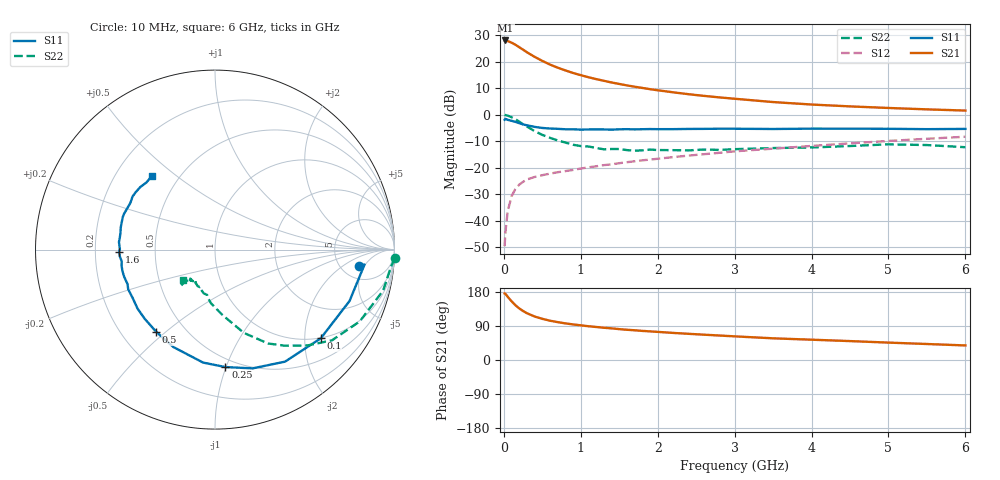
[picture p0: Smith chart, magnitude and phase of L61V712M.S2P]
!  INFINEON TECHNOLOGIES Small Signal Semiconductors
! BFR380L3 , Si-NPN RF-Transistor in TSLP-3-1
!  Vce=1.75 V,  Ic=12.5 mA
! Common Emitter S-Parameters:  07. March 2005
#  GHz  S  MA  R  50
! f  S11  S21  S12  S22
! GHz  Mag  Ang  Mag  Ang  Mag  Ang  Mag  Ang
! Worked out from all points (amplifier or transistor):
!   36 points, 10 MHz to 6 GHz, reference 50 ohm
!   highest |S21| = 28.1 dB at 20 MHz (marker M1)
!   |S21| within 3 dB of that: start of sweep to 224.2 MHz
!   unconditionally stable (mu >= 1): 2.034 GHz to 4.841 GHz
!   at 250 MHz: K = 0.29, MSG = 24.9 dB, |S12| = -25.3 dB
!   at 1.4 GHz: K = 0.91, MSG = 15.5 dB, |S12| = -18.7 dB
!   at 6 GHz: K = 0.97, MSG = 4.9 dB, |S12| = -8.3 dB
!   S11 on the Smith chart (normalised r, x): 10 MHz: 7.23, -3.80; 100 MHz: 0.99, -2.39; 250 MHz: 0.43, -1.00; 500 MHz: 0.35, -0.47; 1.6 GHz: 0.30, -0.01; 6 GHz: 0.36, +0.41
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0.01  0.805 -6.6  25.27 175.6  0.0033 84.4  1.002 -2.8
0.02  0.8373 -5.7  25.29 174.9  0.0059 91.9  0.9845 -5.7
0.05  0.8024 -20.9  24.63 166.9  0.015 81.4  0.9642 -13.7
0.1  0.7691 -40.0  23 155.1  0.0288 70.4  0.9002 -26.4
0.15  0.7361 -58.0  21.05 144.6  0.0397 63.4  0.8248 -37.8
0.2  0.6942 -72.4  18.87 136.1  0.0479 59.1  0.7424 -46.0
0.25  0.6571 -84.9  16.94 129.3  0.0542 54.0  0.6608 -54.1
0.3  0.633 -96.0  15.13 123.5  0.06 51.5  0.6011 -60.5
0.4  0.5903 -113.1  12.41 114.7  0.0668 48.7  0.491 -70.9
0.5  0.5632 -125.5  10.4 108.7  0.0723 47.5  0.4171 -77.2
0.6  0.5496 -135.4  8.864 103.7  0.0773 47.1  0.3667 -83.5
0.7  0.5424 -142.7  7.751 100.0  0.0822 48.0  0.3273 -89.1
0.9  0.5318 -155.4  6.144 93.9  0.0909 49.5  0.2713 -98.4
1.1  0.5279 -163.0  5.11 89.1  0.1018 51.5  0.2515 -104.6
1.4  0.5236 -172.7  4.07 83.5  0.1158 54.1  0.2257 -112.1
1.6  0.5345 -178.6  3.585 79.8  0.127 55.0  0.215 -119.9
2.2  0.535 169.9  2.656 71.5  0.1586 57.9  0.2146 -124.8
2.8  0.5449 160.4  2.129 64.6  0.1911 59.7  0.2171 -131.9
3.5  0.5384 151.2  1.737 57.2  0.2291 59.4  0.2351 -132.4
4.5  0.5456 144.3  1.439 49.9  0.2887 59.4  0.2568 -133.2
5.5  0.5347 135.6  1.264 42.2  0.3519 56.7  0.2679 -134.0
6  0.5405 130.3  1.2 38.4  0.3847 55.0  0.2438 -136.4
